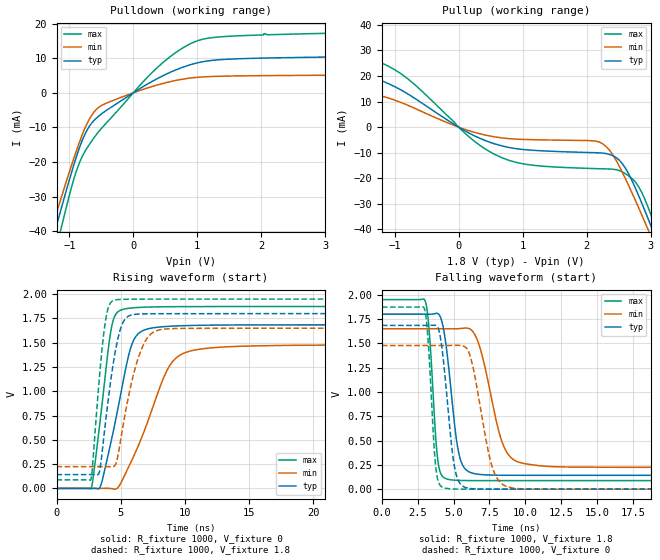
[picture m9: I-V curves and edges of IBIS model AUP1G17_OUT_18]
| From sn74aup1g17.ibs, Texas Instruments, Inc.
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[Model]   AUP1G17_OUT_18
Model_type  Output
Vref =   0
Rref =   1E6
Cref =   30p
Vmeas =   0.9
| variable   typ   min   max
C_comp   2.88pF   2.03pF   4.17pF
| C_pullup   3.17pF   2.03pF   4.17pF
| C_pulldown   2.60pF   2.23pF   3.12pF
[Temperature Range]   40   100   -40
| Ambient temperature   25   85   -40
[Voltage range]   1.8   1.65   1.95
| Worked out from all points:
|   slope of the pulldown table from 0 to 0.27 V, typ, clamps not added: 88.6 ohm
|   slope of the pullup table from 0 to 0.27 V, typ, clamps not added: 73.6 ohm
|   rising waveform, R_fixture 1000, V_fixture 0: 20-80 % time 1.57ns typ, 2.6ns min, 989ps max; typ from 0 V to 1.68 V
|   falling waveform, R_fixture 1000, V_fixture 1.8: 20-80 % time 752ps typ, 1.32ns min, 465ps max; typ from 1.8 V to 0.142 V
|   rising waveform, R_fixture 1000, V_fixture 1.8: 20-80 % time 1.02ns typ, 1.42ns min, 730ps max; typ from 0.142 V to 1.8 V
|   falling waveform, R_fixture 1000, V_fixture 0: 20-80 % time 679ps typ, 1.11ns min, 431ps max; typ from 1.68 V to 0 V
[Pulldown]
| AUP1G17_OUT_18
|   Voltage   I(typ)   I(min)   I(max)
-3.6V     -208.6mA   -189.9mA   -231.7mA
-1.27V    -43.16mA   -39.01mA   -50.14mA
-1.215V   -39.42mA   -35.66mA   -45.88mA
-1.125V   -33.38mA   -30.25mA   -38.97mA
-850mV    -16.31mA   -14.68mA   -20.63mA
-710mV    -10.41mA   -8.408mA   -15.6mA
-555mV    -6.973mA   -4.411mA   -11.55mA
360mV     3.96mA     2.185mA    7.039mA
705mV     6.927mA    3.722mA    12.18mA
1.03V     8.784mA    4.527mA    15.22mA
2.04V     10.05mA    4.966mA    17.1mA
7.2V      11.18mA    5.355mA    18.77mA
[Pullup]
| AUP1G17_OUT_18
|   Voltage   I(typ)   I(min)   I(max)
-3.6V     32.09mA    19.71mA    43.84mA
-3.16V    27.19mA    16.62mA    37.96mA
-2.12V    17.93mA    10.78mA    26.5mA
-1.525V   19.29mA    11.78mA    27.75mA
-1.155V   17.65mA    11.82mA    24.55mA
680mV     -7.373mA   -4.228mA   -12mA
2.185V    -10.05mA   -5.721mA   -16.26mA
2.485V    -12.35mA   -14.1mA    -16.81mA
2.725V    -21.81mA   -26.61mA   -20.47mA
2.94V     -34.55mA   -38.91mA   -30.08mA
3.085V    -43.74mA   -47.5mA    -39.77mA
7.2V      -334.8mA   -315.6mA   -357.6mA
[Ramp]
| AUP1G17_OUT_18
| variable   typ   min   max
dV/dt_r   1.01/1.58E-09   0.89/2.62E-09   1.13/9.93E-10
dV/dt_f   1.00/7.58E-10   0.86/1.33E-09   1.12/4.73E-10
R_load = 1000
[Rising Waveform]
| AUP1G17_OUT_18
R_fixture =   1000
C_fixture =   0
L_fixture =   0
V_fixture =   0
V_fixture_min = 0
V_fixture_max = 0
|   Time   V(typ)   V(min)   V(max)
0s        17.12nV    87.22nV    1.127nV
2.715ns   341.1uV    -27uV      7.153mV
3.42ns    20.07mV    323.8uV    719.5mV
4.22ns    463mV      -759.2uV   1.609V
5.035ns   993.6mV    61.66mV    1.837V
5.735ns   1.426V     252.9mV    1.857V
6.33ns    1.588V     426mV      1.863V
8.605ns   1.668V     1.214V     1.871V
10.12ns   1.677V     1.403V     1.872V
35.9ns    1.685V     1.477V     1.873V
[Falling Waveform]
| AUP1G17_OUT_18
R_fixture =   1000
C_fixture =   0
L_fixture =   0
V_fixture =   1.8
V_fixture_min = 1.65
V_fixture_max = 1.95
|   Time   V(typ)   V(min)   V(max)
0s        1.8V       1.65V      1.95V
3.045ns   1.8V       1.65V      1.926V
3.31ns    1.799V     1.65V      1.611V
3.88ns    1.807V     1.65V      322.1mV
4.495ns   1.457V     1.649V     106.4mV
5.345ns   382.4mV    1.651V     90.17mV
6.31ns    165mV      1.626V     88.23mV
8.375ns   143.3mV    486.9mV    87.9mV
9.56ns    142.5mV    276.8mV    87.9mV
35.9ns    142.2mV    224.7mV    87.89mV
[Rising Waveform]
| AUP1G17_OUT_18
R_fixture =   1000
C_fixture =   0
L_fixture =   0
V_fixture =   1.8
V_fixture_min = 1.65
V_fixture_max = 1.95
|   Time   V(typ)   V(min)   V(max)
0s        142.2mV    224.7mV    87.89mV
2.69ns    142.5mV    224.7mV    98.55mV
3.33ns    165mV      224.9mV    1.123V
3.705ns   549.5mV    224.8mV    1.62V
4.03ns    913.7mV    224.1mV    1.859V
4.45ns    1.31V      225.7mV    1.936V
5.19ns    1.711V     649.4mV    1.948V
6.32ns    1.795V     1.322V     1.949V
7.83ns    1.799V     1.626V     1.95V
35.9ns    1.8V       1.65V      1.95V
[Falling Waveform]
| AUP1G17_OUT_18
R_fixture =   1000
C_fixture =   0
L_fixture =   0
V_fixture =   0
V_fixture_min = 0
V_fixture_max = 0
|   Time   V(typ)   V(min)   V(max)
0s        1.685V     1.478V     1.873V
2.965ns   1.684V     1.477V     1.857V
3.755ns   1.684V     1.477V     231.4mV
4.3ns     1.311V     1.478V     14.99mV
4.925ns   366.4mV    1.479V     2.232mV
5.34ns    85.24mV    1.479V     661.8uV
6.2ns     6.153mV    1.345V     71.16uV
7.74ns    225.1uV    206.9mV    4.025uV
8.785ns   46.88uV    22.37mV    791.7nV
35.9ns    -43.81nV   22.97nV    -18.58nV
